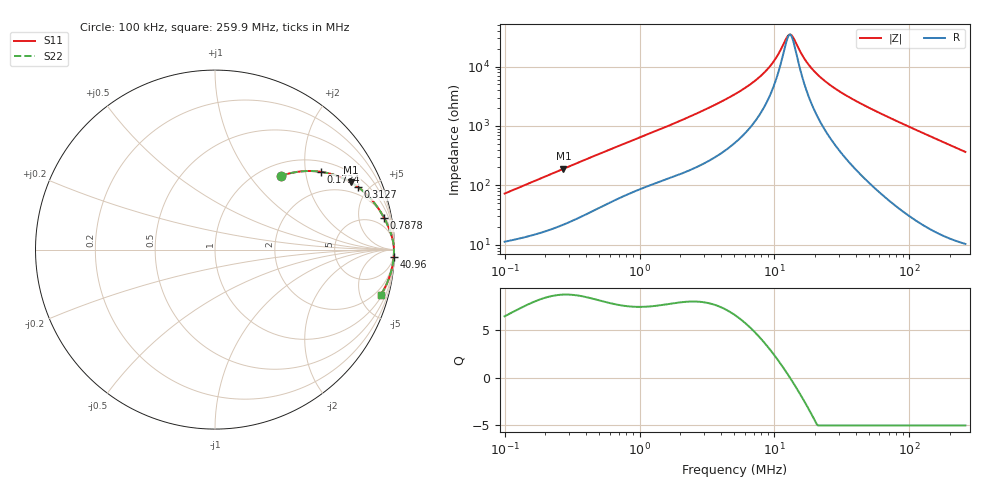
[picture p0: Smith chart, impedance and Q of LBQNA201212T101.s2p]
! LBQNA201212T101  S-PARAMETER MODEL  ( General Type )
! Model Generated by TAIYO YUDEN Corporation (http://www.ty-top.com)
! Version 1.0
! TAIYO YUDEN Control No. 191025NI43SB-FBB
! Copyright(c) 2019 TAIYO YUDEN CO.,LTD. All Rights Reserved.
! Product Description (link to TY-COMPAS)
! https://ds.yuden.co.jp/TYCOMPAS/or/detail?pn=LBQNA201212T101K&u=M
! Products Name : Inductors
! Characteristics :
!  Inductance : 100 uH , SRF(min) : 8.0 MHz , DC Resistance(max) : 9.1 Ohm
!  Rated Current : Saturation :60 mA , Temp Rise : 100 mA (20 degC)
!  Case Size : 2.0 x 1.25 / 0.079 x 0.049 [mm/inch] , Thickness : 1.25 / 0.049 [mm/inch]
!  (Conditions: Temperature = 25 degC , DC Bias Current/Voltage = 0A / 0V)
! External Node Assignments :
!  1  o---GGG---o  2
! GND o---------o GND
! Frequency Range : 0.1MHz  -  259.929867MHz  [ 402 STEP ]
# MHz S RI R 50
! Freq[MHz].  S11 Real  S11 Imag  S21 Real  S21 Imag  S12 Real  S12 Imag  S22 Real  S22 Imag
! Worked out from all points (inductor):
!   401 points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, 100 kHz to 259.9 MHz, reference 50 ohm
!   read as one part in series: L = 113 uH near 104 kHz
!   highest Q = 8.65 at 272.5 kHz (marker M1), where L = 110 uH
!   self-resonance near 12.84 MHz
!   S11 on the Smith chart (normalised r, x): 100 kHz: 1.23, +1.44; 173.4 kHz: 1.30, +2.44; 312.7 kHz: 1.50, +4.30; 787.8 kHz: 2, +10; 40.96 MHz: 4, -51; 259.9 MHz: 1.21, -7.31
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0.1  0.3657 0.4097  0.6343 -0.4097  0.6343 -0.4097  0.3657 0.4097
0.173396  0.5908 0.4333  0.4092 -0.4333  0.4092 -0.4333  0.5908 0.4333
0.272517  0.7583 0.3742  0.2417 -0.3742  0.2417 -0.3742  0.7583 0.3742
0.312719  0.7981 0.3477  0.2019 -0.3477  0.2019 -0.3477  0.7981 0.3477
0.37324  0.8408 0.3117  0.1592 -0.3117  0.1592 -0.3117  0.8408 0.3117
0.787771  0.9412 0.1776  0.0588 -0.1776  0.0588 -0.1776  0.9412 0.1776
1.393082  0.9725 0.11  0.0275 -0.11  0.0275 -0.11  0.9725 0.11
2.940276  0.9901 0.054  0.00988 -0.054  0.00988 -0.054  0.9901 0.054
5.098332  0.9948 0.0286  0.00523 -0.0286  0.00523 -0.0286  0.9948 0.0286
6.846761  0.996 0.0183  0.00402 -0.0183  0.00402 -0.0183  0.996 0.0183
8.668239  0.9966 0.0112  0.00342 -0.0112  0.00342 -0.0112  0.9966 0.0112
10.14444  0.9969 0.00676  0.00314 -0.00676  0.00314 -0.00676  0.9969 0.00676
12.10772  0.9971 0.00192  0.00294 -0.00192  0.00294 -0.00192  0.9971 0.00192
12.84321  0.9971 0.000326  0.00289 -0.000326  0.00289 -0.000326  0.9971 0.000326
13.62339  0.9972 -0.00127  0.00285 0.00127  0.00285 0.00127  0.9972 -0.00127
16.25996  0.9972 -0.00613  0.00279 0.00613  0.00279 0.00613  0.9972 -0.00613
19.02902  0.9972 -0.0106  0.0028 0.0106  0.0028 0.0106  0.9972 -0.0106
26.06218  0.997 -0.0205  0.00305 0.0205  0.00305 0.0205  0.997 -0.0205
40.96048  0.9959 -0.0386  0.00413 0.0386  0.00413 0.0386  0.9959 -0.0386
71.02397  0.992 -0.0716  0.00804 0.0716  0.00804 0.0716  0.992 -0.0716
138.5695  0.9757 -0.1408  0.0243 0.1408  0.0243 0.1408  0.9757 -0.1408
259.9299  0.9242 -0.2508  0.0758 0.2508  0.0758 0.2508  0.9242 -0.2508
